FUNCTION_BLOCK FB_UpdateProduct
VAR_IN_OUT
	fbClient:FB_IotHttpClient;
END_VAR
VAR_OUTPUT
	bBusy:BOOL;
	bError:BOOL;
	
END_VAR
VAR
	fbRequest			: FB_IotHttpRequest;
	fbJsonSend				: FB_JsonDomParser;
	jsonDoc				: SJsonValue;
	nState				: UDINT;
	AddRisingEdge			: R_TRIG;
	fbGetProductByBarCode:FB_GetProductByBarCode;
//	domParse:FB_JsonDomParser;
	
END_VAR
//HMI
VAR
	bSend:BOOL;
	nStatusCode:UINT;
	product:ST_Product;
END_VAR

AddRisingEdge(CLK:=bSend , Q=> );
CASE nState OF
	0:
		IF AddRisingEdge.Q AND product.BarCode<>'' THEN
			nStatusCode:=0;
			nState:=10;
			bBusy:=TRUE;
			bError:=FALSE;
		END_IF
	
	10:
		
		jsonDoc:=fbJsonSend.NewDocument();
		fbJsonSend.AddInt64Member(jsonDoc,'id',0);
		fbJsonSend.AddStringMember(jsonDoc,'barCode',product.BarCode);
		fbJsonSend.AddDoubleMember(jsonDoc,'finalPressure',product.FinalPressure);
		fbJsonSend.AddDoubleMember(jsonDoc,'finalDisplacement',product.FinalDisplacement);
		fbJsonSend.AddBoolMember(jsonDoc,'isQualified',product.IsQualified);
		IF fbRequest.SendJsonDomRequest(sUri:='/Product',fbClient:=fbClient,eRequestType:=ETcIotHttpRequestType.HTTP_PUT,fbJson:=fbJsonSend,0) THEN
			nState:=20;
		END_IF
	20:
		IF NOT fbRequest.bBusy THEN
			nStatusCode:=fbRequest.nStatusCode;
			IF nStatusCode=200 THEN
				product.BarCode:='';
			END_IF
			nState:=100;
		END_IF
			
	100:
		bBusy:=FALSE;
		nState:=0;
END_CASE

END_FUNCTION_BLOCK
